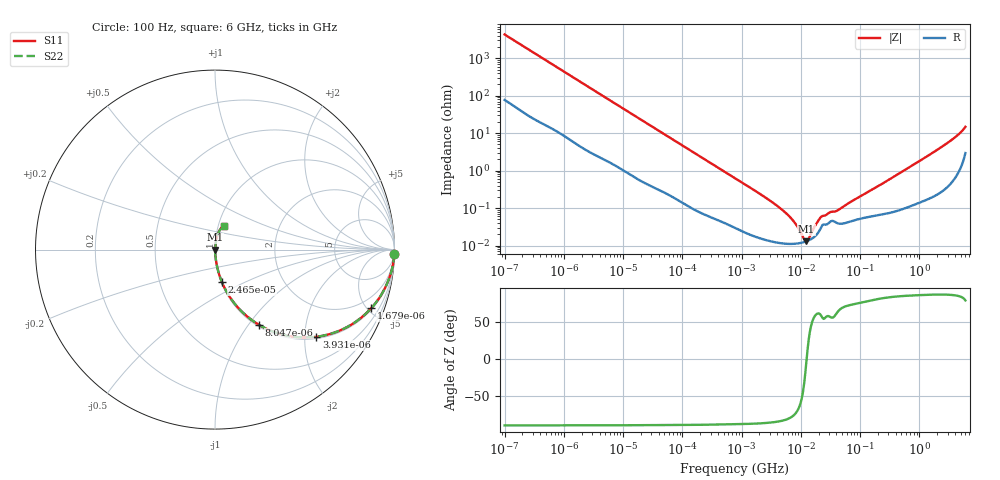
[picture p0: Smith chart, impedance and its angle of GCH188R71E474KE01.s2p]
!Murata Part Number: GCH188R71E474KE01
!These Parameters are Measured in Series Mode Connection
!Data Generated on Jun 19, 2026
!  o--ll--o
!Port1  Port2
!  o------o
!Operation Temp=25[degC], DC Bias Voltage=0[V]
!Freq. Start=100[Hz] Stop=6[GHz] 401[Steps]
# Hz S RI R 50
!Freq.(Hz) S11(Real) S11(Imag) S21(Real) S21(Imag) S12(Real) S12(Imag) S22(Real) S22(Imag)
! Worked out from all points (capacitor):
!   401 points, 100 Hz to 6 GHz, reference 50 ohm
!   read as one part in series: C = 368 nF near 109 Hz
!   lowest |Z| = 13 mohm at 12.44 MHz (marker M1)
!   series resonance near 12.54 MHz, so ESL is about 440 pH
!   S11 on the Smith chart (normalised r, x): 100 Hz: 3, -86; 1.679 kHz: 1.10, -5.30; 3.931 kHz: 1.05, -2.28; 8.047 kHz: 1.03, -1.13; 24.65 kHz: 1.01, -0.37; 6 GHz: 1.06, +0.29
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100  0.999 -0.0232  0.000952 0.0232  0.000952 0.0232  0.999 -0.0232
501  0.9851 -0.1124  0.0149 0.1124  0.0149 0.1124  0.9851 -0.1124
1679  0.8708 -0.3262  0.1292 0.3262  0.1292 0.3262  0.8708 -0.3262
2008  0.8268 -0.3692  0.1732 0.3692  0.1732 0.3692  0.8268 -0.3692
3931  0.5648 -0.4858  0.4352 0.4858  0.4352 0.4858  0.5648 -0.4858
8047  0.2461 -0.4197  0.7539 0.4197  0.7539 0.4197  0.2461 -0.4197
13169  0.1129 -0.3054  0.8871 0.3054  0.8871 0.3054  0.1129 -0.3054
24648  0.0377 -0.179  0.9623 0.179  0.9623 0.179  0.0377 -0.179
40335  0.016 -0.1128  0.984 0.1128  0.984 0.1128  0.016 -0.1128
129199  0.00243 -0.0366  0.9976 0.0366  0.9976 0.0366  0.00243 -0.0366
774597  0.000336 -0.00632  0.9997 0.00632  0.9997 0.00632  0.000336 -0.00632
5079039  0.000114 -0.00084  0.9999 0.00084  0.9999 0.00084  0.000114 -0.00084
7599586  0.000112 -0.000428  0.9999 0.000428  0.9999 0.000428  0.000112 -0.000428
1.137099e7  0.000124 -8.1e-05  0.9999 8.1e-05  0.9999 8.1e-05  0.000124 -8.1e-05
1.243624e7  0.00013 -6.9e-06  0.9999 6.9e-06  0.9999 6.9e-06  0.00013 -6.9e-06
1.360128e7  0.000138 6.79e-05  0.9999 -6.79e-05  0.9999 -6.79e-05  0.000138 6.79e-05
1.555665e7  0.000155 0.000183  0.9998 -0.000183  0.9998 -0.000183  0.000155 0.000183
2.225763e7  0.000318 0.000501  0.9997 -0.000501  0.9997 -0.000501  0.000318 0.000501
4.165952e7  0.000396 0.000772  0.9996 -0.000772  0.9996 -0.000772  0.000396 0.000772
3.124326e8  0.000773 0.00578  0.9992 -0.00578  0.9992 -0.00578  0.000773 0.00578
2.562649e9  0.00509 0.046  0.9949 -0.046  0.9949 -0.046  0.00509 0.046
6e9  0.0474 0.1338  0.9526 -0.1338  0.9526 -0.1338  0.0474 0.1338
